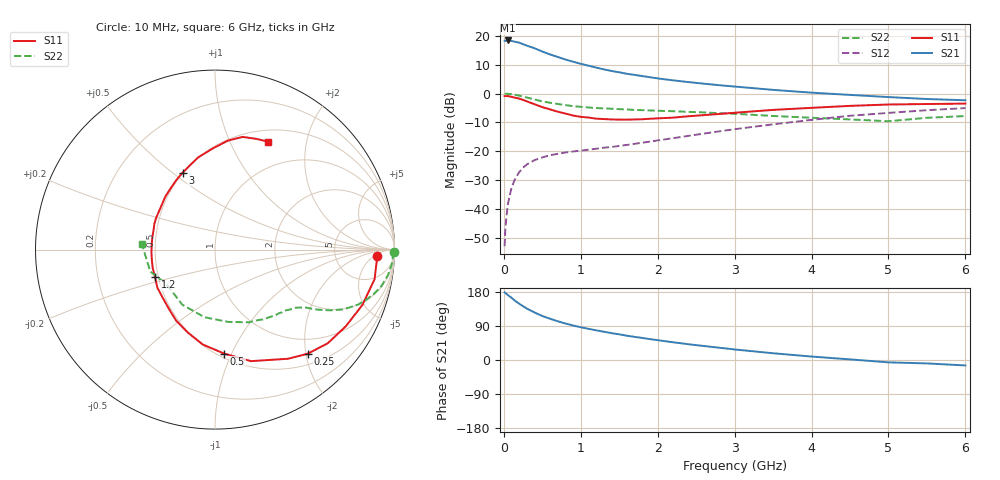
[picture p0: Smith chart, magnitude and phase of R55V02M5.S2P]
! SIEMENS Small Signal Semiconductors
! BFR183
! Si NPN RF Bipolar Junction Transistor in SOT23
! VCE = 5 V  IC = 2.5 mA
! Common Emitter S-Parameters:  May  1996
# GHz  S  MA  R  50
!  f  S11  S21  S12  S22
! GHz  MAG  ANG  MAG  ANG  MAG  ANG  MAG  ANG
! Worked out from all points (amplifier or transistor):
!   36 points, 10 MHz to 6 GHz, reference 50 ohm
!   highest |S21| = 18.4 dB at 50 MHz (marker M1)
!   |S21| within 3 dB of that: start of sweep to 426.3 MHz
!   unconditionally stable (mu >= 1): 1.33 GHz to 2.81 GHz
!   at 250 MHz: K = 0.26, MSG = 21.3 dB, |S12| = -25.6 dB
!   at 1.4 GHz: K = 1.03, MAG = 12.1 dB, |S12| = -18.5 dB
!   at 6 GHz: K = 0.89, MSG = 1.4 dB, |S12| = -5.0 dB
!   S11 on the Smith chart (normalised r, x): 10 MHz: 18, -6; 250 MHz: 0.70, -2.04; 500 MHz: 0.54, -0.94; 1.2 GHz: 0.48, -0.17; 3 GHz: 0.50, +0.54; 6 GHz: 0.64, +1.40
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0.01  0.9045 -2.1  8.162 178.6  0.0023 93.8  0.9949 -0.8
0.02  0.9031 -4.2  8.108 176.6  0.0048 86.6  0.9924 -1.7
0.05  0.9044 -10.5  8.271 171.8  0.0118 84.4  0.9898 -4.3
0.1  0.8771 -20.6  8.103 164.1  0.0237 79.2  0.9739 -8.5
0.15  0.8449 -30.3  7.826 155.6  0.0342 72.7  0.9496 -12.3
0.2  0.8168 -39.7  7.579 148.5  0.0439 68.8  0.9189 -15.6
0.25  0.7767 -48.3  7.12 141.9  0.0525 64.3  0.8856 -18.6
0.3  0.7318 -56.2  6.727 135.7  0.0596 61.4  0.8542 -21.0
0.4  0.6531 -72.1  6.059 125.3  0.0707 55.3  0.7904 -24.9
0.5  0.582 -84.9  5.32 116.1  0.0787 51.5  0.7325 -27.5
0.6  0.5329 -97.4  4.743 108.9  0.0859 48.9  0.6928 -29.1
0.8  0.4511 -118.7  3.875 96.3  0.0957 46.0  0.6303 -31.5
0.9  0.4166 -128.4  3.547 91.0  0.0996 46.4  0.6061 -32.3
1.1  0.3848 -146.5  3.029 82.3  0.1069 47.1  0.5741 -34.3
1.2  0.368 -155.2  2.811 78.3  0.111 47.6  0.5621 -35.1
1.6  0.3541 175.5  2.195 64.1  0.1294 50.5  0.53 -39.3
2.2  0.3833 142.1  1.691 46.8  0.1691 54.4  0.4951 -48.0
3  0.4652 112.9  1.321 27.8  0.242 53.4  0.4472 -64.9
3.5  0.5216 100.5  1.157 17.8  0.2934 49.4  0.4094 -79.7
4.5  0.6121 83.1  0.947 1.6  0.4129 38.0  0.3569 -120.7
5.5  0.6589 69.4  0.804 -9.0  0.5152 24.3  0.3808 -161.3
6  0.6697 63.9  0.765 -14.4  0.5604 15.4  0.408 175.9
